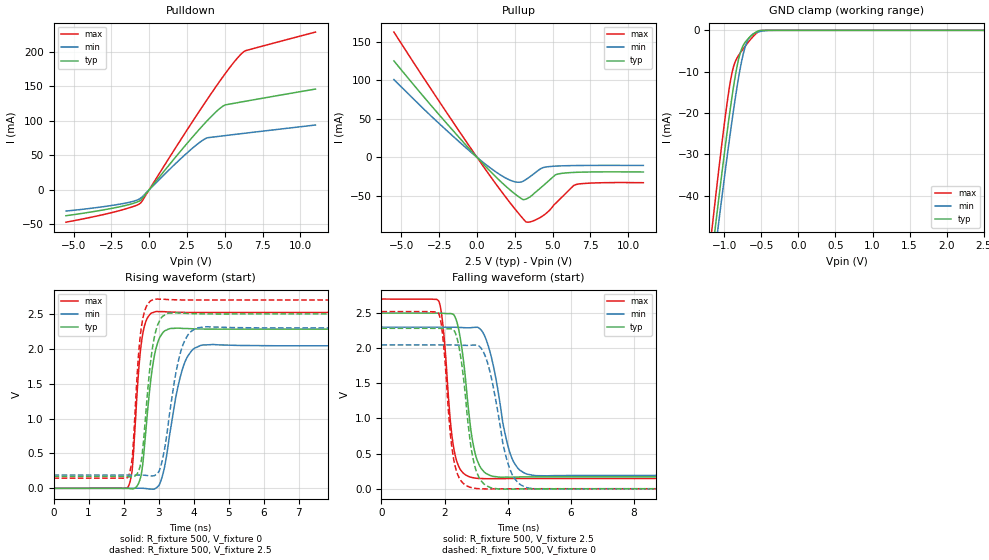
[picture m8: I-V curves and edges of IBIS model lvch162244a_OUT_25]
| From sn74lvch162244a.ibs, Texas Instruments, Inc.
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[Model]   lvch162244a_OUT_25
Model_type  3-state
Enable   Active-Low
Vref =   0
Rref =   500
Cref =   30p
Vmeas =   1.25
| variable   typ   min   max
C_comp   4.95pF   4.44pF   5.95pF
| C_pullup   3.08pF   2.22pF   5.35pF
| C_pulldown   3.30pF   2.54pF   5.10pF
| C_tri-state   4.95pF   4.44pF   5.95pF
[Temperature Range]   40   100   -40
| Ambient temperature   25   85   -40
[Voltage range]   2.5   2.3   2.7
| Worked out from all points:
|   slope of the pulldown table from 0 to 0.375 V, typ, clamps not added: 36.5 ohm
|   slope of the pullup table from 0 to 0.375 V, typ, clamps not added: 47.7 ohm
|   GND clamp passes 1 mA (typ) near -0.61 V on its own axis
|   rising waveform, R_fixture 500, V_fixture 0: 20-80 % time 283ps typ, 432ps min, 209ps max; typ from 0 V to 2.28 V
|   falling waveform, R_fixture 500, V_fixture 2.5: 20-80 % time 369ps typ, 527ps min, 285ps max; typ from 2.5 V to 0.17 V
|   rising waveform, R_fixture 500, V_fixture 2.5: 20-80 % time 270ps typ, 403ps min, 199ps max; typ from 0.17 V to 2.5 V
|   falling waveform, R_fixture 500, V_fixture 0: 20-80 % time 362ps typ, 523ps min, 282ps max; typ from 2.28 V to 0 V
[GND Clamp]
| lvch162244a_OUT_25
|   Voltage   I(typ)   I(min)   I(max)
-5.5V     -768.1mA   -753.5mA   -792mA
-1.175V   -56.09mA   -61.39mA   -49.74mA
-1.12V    -47.75mA   -53.28mA   -41.03mA
-1.095V   -44mA      -49.63mA   -37.13mA
-1.07V    -40.29mA   -46.01mA   -33.28mA
-955mV    -23.91mA   -29.87mA   -16.84mA
-885mV    -14.93mA   -20.68mA   -9.567mA
-810mV    -7.325mA   -11.87mA   -6.191mA
-740mV    -3.547mA   -5.51mA    -4.383mA
-620mV    -1.086mA   -1.003mA   -1.699mA
-475mV    -10.23uA   -143.8uA   -14uA
2.5V      50.35pA    32.01nA    -2.079nA
[Pulldown]
| lvch162244a_OUT_25
|   Voltage   I(typ)   I(min)   I(max)
-5.5V     -37.53mA   -30.77mA   -46.9mA
-2.025V   -24.95mA   -21.12mA   -30.54mA
-1.07V    -19.77mA   -16.78mA   -24.35mA
-595mV    -15.6mA    -12.59mA   -19.64mA
2.135V    57.37mA    45.87mA    73.9mA
3.565V    93.41mA    71.92mA    121.7mA
3.885V    100.9mA    75.32mA    132.1mA
4.915V    121.4mA    78.09mA    164.5mA
5.595V    125mA      79.88mA    184.2mA
6.09V     127mA      81.17mA    196.4mA
6.4V      128.2mA    81.97mA    201.4mA
11V       145.7mA    93.67mA    228.1mA
[Pullup]
| lvch162244a_OUT_25
|   Voltage   I(typ)   I(min)   I(max)
-5.5V     125mA      100.8mA    162.3mA
-2.285V   50.2mA     39.84mA    66.07mA
780mV     -16.14mA   -12.22mA   -21.79mA
2.345V    -44.85mA   -30.73mA   -62.84mA
3.02V     -54.49mA   -31.12mA   -78.94mA
3.23V     -54.01mA   -28.69mA   -83.44mA
3.6V      -49.73mA   -23.57mA   -83.08mA
4.24V     -38.91mA   -14.33mA   -77.14mA
4.705V    -30.92mA   -12.08mA   -70.17mA
5.19V     -22.63mA   -11.31mA   -59.63mA
6.52V     -19.37mA   -10.56mA   -35.37mA
11V       -18.92mA   -10.44mA   -32.8mA
[Ramp]
| lvch162244a_OUT_25
| variable   typ   min   max
dV/dt_r   1.38/2.95E-10   1.24/4.48E-10   1.52/2.16E-10
dV/dt_f   1.40/3.73E-10   1.27/5.45E-10   1.53/2.89E-10
R_load = 500
[Rising Waveform]
| lvch162244a_OUT_25
R_fixture =   500
C_fixture =   0
L_fixture =   0
V_fixture =   0
V_fixture_min = 0
V_fixture_max = 0
|   Time   V(typ)   V(min)   V(max)
0s        581.4pV    1.823nV    17.86nV
2.125ns   -954.5uV   233.7uV    15.18mV
2.25ns    -8.833mV   904.6uV    281.7mV
2.535ns   292.2mV    980.8uV    2.171V
2.765ns   1.495V     -10.64mV   2.499V
2.935ns   2.019V     6.141mV    2.534V
3.16ns    2.251V     275.2mV    2.533V
3.7ns     2.292V     1.734V     2.522V
4.28ns    2.284V     2.057V     2.521V
40ns      2.283V     2.044V     2.521V
[Falling Waveform]
| lvch162244a_OUT_25
R_fixture =   500
C_fixture =   0
L_fixture =   0
V_fixture =   2.5
V_fixture_min = 2.3
V_fixture_max = 2.7
|   Time   V(typ)   V(min)   V(max)
0s        2.5V       2.3V       2.7V
1.82ns    2.499V     2.3V       2.668V
1.95ns    2.497V     2.3V       2.317V
2.295ns   2.475V     2.299V     564mV
2.52ns    2.079V     2.295V     260.2mV
2.985ns   471.8mV    2.298V     150.5mV
3.43ns    191mV      1.962V     143mV
4.12ns    165.1mV    448mV      145.2mV
4.83ns    169.1mV    189.3mV    145.8mV
40ns      169.9mV    189.8mV    145.7mV
[Rising Waveform]
| lvch162244a_OUT_25
R_fixture =   500
C_fixture =   0
L_fixture =   0
V_fixture =   2.5
V_fixture_min = 2.3
V_fixture_max = 2.7
|   Time   V(typ)   V(min)   V(max)
0s        169.9mV    189.7mV    145.7mV
2.125ns   168.8mV    190mV      161.8mV
2.25ns    161mV      190.6mV    447.5mV
2.525ns   459mV      190.4mV    2.36V
2.76ns    1.756V     178.8mV    2.681V
2.93ns    2.271V     198.2mV    2.712V
3.135ns   2.472V     464.3mV    2.711V
3.665ns   2.511V     2.01V      2.701V
4.3ns     2.501V     2.314V     2.7V
40ns      2.5V       2.3V       2.7V
[Falling Waveform]
| lvch162244a_OUT_25
R_fixture =   500
C_fixture =   0
L_fixture =   0
V_fixture =   0
V_fixture_min = 0
V_fixture_max = 0
|   Time   V(typ)   V(min)   V(max)
0s        2.284V     2.047V     2.522V
1.82ns    2.283V     2.047V     2.489V
1.95ns    2.281V     2.047V     2.132V
2.295ns   2.257V     2.046V     401.4mV
2.505ns   1.89V      2.043V     122.2mV
2.985ns   276.2mV    2.045V     4.954mV
3.39ns    28.81mV    1.747V     -2.951mV
4.095ns   -5.341mV   247.9mV    -508.7uV
4.84ns    -1.055mV   -1.43mV    100.2uV
40ns      16.75uV    45.77uV    5.83uV
